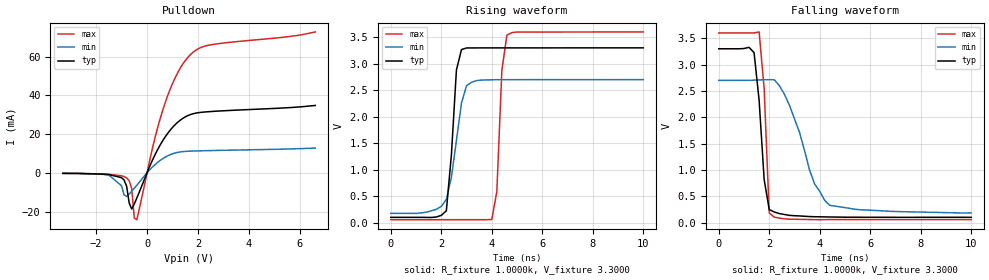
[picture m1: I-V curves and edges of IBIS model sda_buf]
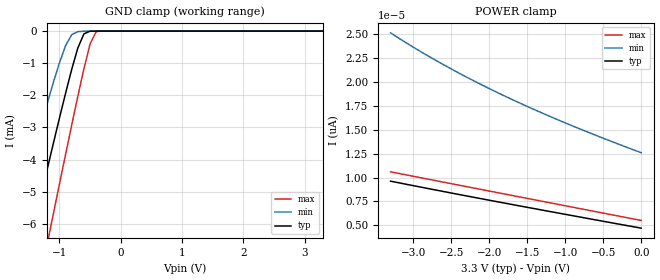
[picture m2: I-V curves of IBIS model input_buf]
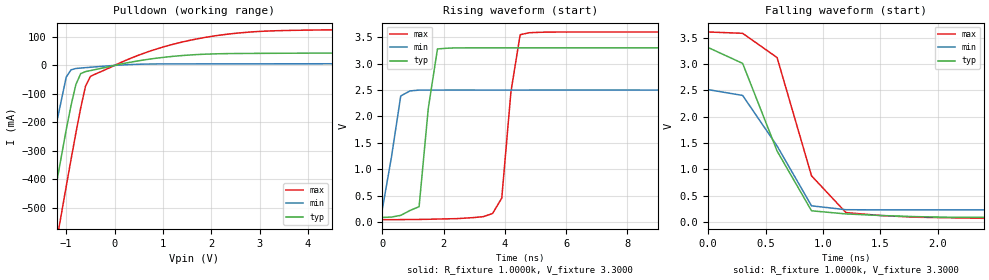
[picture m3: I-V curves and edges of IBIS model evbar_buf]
| IBIS file stts424.ibs created by s2ibis2 version 1.1
| North Carolina State University Electronics Research Laboratory  1995
[IBIS ver]   2.1
[File name]   stts424.ibs
[File Rev]   1.0
[Date]   Jul 30, 2008
[Source]   ST models
[Copyright]   ST Microelectronics Inc.
|   Component stts424E02 [Package]
[Component]   STTS424E02
|[Package]
[Manufacturer]   ST Microelectronics
[Package]
| variable   typ   min   max
R_pkg   45.0000m   42.0000m   47.0000m
L_pkg   0.6300nH   0.5700nH   0.6600nH
C_pkg   59.0000fF   44.0000fF   62.0000fF
[Pin]  signal_name   model_name   R_pin   L_pin   C_pin
| evbardummy   dummy
| EN   dummy   dummy
| rdlowdummy   dummy
1   A0   input_buf
2   A1   input_buf
3   A2   input_buf
4   vss   GND
5   sda   sda_buf
6   SCL   input_buf
7   EVENT#   evbar_buf
8   vcc   POWER
| Models and submodels in the file (3): sda_buf (Open_drain), input_buf (Input), evbar_buf (Open_drain)
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|   Model sda_buf
[Model]   sda_buf
Model_type   Open_drain
Polarity   Inverting
Enable   Active-High
Vmeas =   1.5000V
Cref =1.000e-10F
Rref =   0.6430k
Vref =   1.7500V
C_comp   1.0500pF   1.0300pF   1.0600pF
[Temperature Range]   27.0000   0.1250k   -55.0000
[Voltage Range]   3.3000V   2.7000V   3.6000V
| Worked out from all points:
|   slope of the pulldown table from 0 to 0.495 V, typ, clamps not added: 35.7 ohm
|   rising waveform, R_fixture 1.0000k, V_fixture 3.3000: 20-80 % time 274ps typ, 466ps min, 189ps max; typ from 0.1 V to 3.3 V
|   falling waveform, R_fixture 1.0000k, V_fixture 3.3000: 20-80 % time 302ps typ, 1.04ns min, 215ps max; typ from 3.3 V to 0.1 V
[Pulldown]
| voltage   I(typ)   I(min)   I(max)
-3.3V     -200uA     -300uA     -300uA
-1.5V     -890uA     -1.1mA     -730uA
-800mV    -6.876mA   -12.11mA   -2.6mA
-600mV    -18.68mA   -9.462mA   -8.186mA
-500mV    -16.04mA   -7.947mA   -23.29mA
-400mV    -12.96mA   -6.399mA   -24.16mA
200mV     6.187mA    2.845mA    12.01mA
700mV     18.29mA    8.01mA     35.72mA
1.2V      26.06mA    10.56mA    51.61mA
1.7V      30.05mA    11.2mA     60.96mA
2.5V      31.63mA    11.49mA    66.03mA
6.6V      34.77mA    12.78mA    72.67mA
[Ramp]
| variable   typ   min   max
dV/dt_r   0.9137/0.3881n   0.3403/0.9150n   1.4872/0.2325n
dV/dt_f   0.9113/1.3748n   0.3362/3.2715n   1.4872/0.5289n
R_load = 50.0000
[Rising Waveform]
R_fixture = 1.0000k
V_fixture = 3.3000
V_fixture_min = 2.7000
V_fixture_max = 3.6000
| time   V(typ)   V(min)   V(max)
0s        100.2mV    175.7mV    56.38mV
2.2ns     223.3mV    437.5mV    56.38mV
2.4ns     1.279V     856.6mV    56.38mV
2.6ns     2.885V     1.553V     56.38mV
2.8ns     3.267V     2.258V     56.38mV
4ns       3.299V     2.697V     58.97mV
4.2ns     3.299V     2.699V     583.9mV
4.4ns     3.299V     2.699V     2.876V
4.6ns     3.299V     2.699V     3.541V
10ns      3.3V       2.7V       3.6V
[Falling Waveform]
R_fixture = 1.0000k
V_fixture = 3.3000
V_fixture_min = 2.7000
V_fixture_max = 3.6000
| time   V(typ)   V(min)   V(max)
0s        3.3V       2.7V       3.6V
1.4ns     3.226V     2.704V     3.601V
1.6ns     2.323V     2.708V     3.619V
1.8ns     816.7mV    2.712V     2.543V
2ns       249.3mV    2.712V     183.9mV
2.2ns     201mV      2.711V     102.8mV
2.8ns     137.2mV    2.23V      64.17mV
3.8ns     111.4mV    732.4mV    55.59mV
4.4ns     106.2mV    327.4mV    56.72mV
10ns      100.1mV    183.2mV    56.38mV
|   Model input_buf
[Model]   input_buf
Model_type   Input
Vinl =   0.3000V
Vinh =   0.7000V
C_comp   3.2900pF   3.2200pF   4.6400pF
[Temperature Range]   27.0000   0.1250k   -55.0000
[Voltage Range]   3.3000V   2.7000V   3.6000V
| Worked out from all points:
|   GND clamp passes 1 mA (typ) near -0.77 V on its own axis
[GND_clamp]
| voltage   I(typ)   I(min)   I(max)
-3.3V     -21.76mA   -17.32mA   -26.61mA
-1.8V     -9.225mA   -6.439mA   -12.3mA
-1.5V     -6.749mA   -4.315mA   -9.457mA
-1.4V     -5.929mA   -3.619mA   -8.513mA
-1.2V     -4.303mA   -2.257mA   -6.631mA
-1.1V     -3.5mA     -1.603mA   -5.695mA
-900mV    -1.935mA   -454.4uA   -3.84mA
-700mV    -526.2uA   -17.75uA   -2.029mA
-600mV    -85.3uA    -3.97uA    -1.166mA
-500mV    -3.274uA   -1.013uA   -397.5uA
-400mV    -125.8nA   -249.8nA   -16.01uA
3.3V      4.712pA    14.41pA    5.057pA
[POWER_clamp]
| voltage   I(typ)   I(min)   I(max)
-3.3V     9.621pA    25.1pA     10.59pA
-3V       9.15pA     23.61pA    10.13pA
-2.6V     8.535pA    21.77pA    9.511pA
-2.3V     8.079pA    20.49pA    9.05pA
-1.9V     7.479pA    18.9pA     8.434pA
-1.5V     6.888pA    17.42pA    7.819pA
-1V       6.156pA    15.7pA     7.051pA
-500mV    5.431pA    14.1pA     6.284pA
0V        4.712pA    12.59pA    5.517pA
|   Model evbar_buf
[Model]   evbar_buf
Model_type   Open_drain
Polarity   Inverting
Enable   Active-Low
Vmeas =   1.5000V
Rref =   0.6430k
Vref =   1.7500V
C_comp   1.0300pF   1.0100pF   1.0500pF
[Temperature Range]   27.0000   0.1250k   -55.0000
[Voltage Range]   3.3000V   2.7000V   3.6000V
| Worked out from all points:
|   slope of the pulldown table from 0 to 0.495 V, typ, clamps not added: 30.7 ohm
|   rising waveform, R_fixture 1.0000k, V_fixture 3.3000: 20-80 % time 364ps typ, 376ps min, 372ps max; typ from 0.086 V to 3.3 V
|   falling waveform, R_fixture 1.0000k, V_fixture 3.3000: 20-80 % time 401ps typ, 391ps min, 321ps max; typ from 3.31 V to 0.088 V
[Pulldown]
| voltage   I(typ)   I(min)   I(max)
-3.3V     -2.461A    -2.191A    -2.689A
-1.7V     -888.1mA   -634.3mA   -1.106A
-1.5V     -694.7mA   -446.6mA   -909.8mA
-1V       -226.1mA   -41.11mA   -425.3mA
-900mV    -140.7mA   -15.42mA   -330.6mA
-800mV    -67.39mA   -10.86mA   -238mA
-700mV    -28.76mA   -9.172mA   -149.4mA
-600mV    -21.76mA   -7.767mA   -72.8mA
-500mV    -18.21mA   -6.436mA   -38.52mA
600mV     19mA       4.492mA    42.33mA
2.7V      42.06mA    5.607mA    115.9mA
6.6V      45.16mA    6.405mA    128.4mA
[Ramp]
| variable   typ   min   max
dV/dt_r   1.0793/0.7716n   0.1669/0.3467n   1.6634/1.4848n
dV/dt_f   1.0793/0.8139n   0.1669/0.2970n   1.6634/1.4233n
R_load = 50.0000
[Rising Waveform]
R_fixture = 1.0000k
V_fixture = 3.3000
V_fixture_min = 2.5000
V_fixture_max = 3.6000
| time   V(typ)   V(min)   V(max)
0s        86mV       242.9mV    43.79mV
600ps     125.5mV    2.388V     45.39mV
1.2ns     290.4mV    2.499V     48.47mV
1.5ns     2.153V     2.5V       51.6mV
1.8ns     3.278V     2.499V     56.07mV
3.3ns     3.299V     2.5V       101.6mV
3.9ns     3.299V     2.499V     452.7mV
4.2ns     3.299V     2.499V     2.469V
4.5ns     3.299V     2.5V       3.548V
15ns      3.3V       2.5V       3.6V
[Falling Waveform]
R_fixture = 1.0000k
V_fixture = 3.3000
V_fixture_min = 2.5000
V_fixture_max = 3.6000
| time   V(typ)   V(min)   V(max)
0s        3.31V      2.512V     3.606V
300ps     3.01V      2.402V     3.58V
600ps     1.347V     1.443V     3.12V
900ps     213.1mV    307.7mV    876.4mV
1.2ns     153.7mV    233.7mV    178.7mV
1.5ns     124.2mV    230.9mV    123.8mV
1.8ns     102.4mV    231.3mV    91.66mV
3.9ns     88.01mV    231.1mV    52.1mV
15ns      88mV       230.7mV    44.5mV
